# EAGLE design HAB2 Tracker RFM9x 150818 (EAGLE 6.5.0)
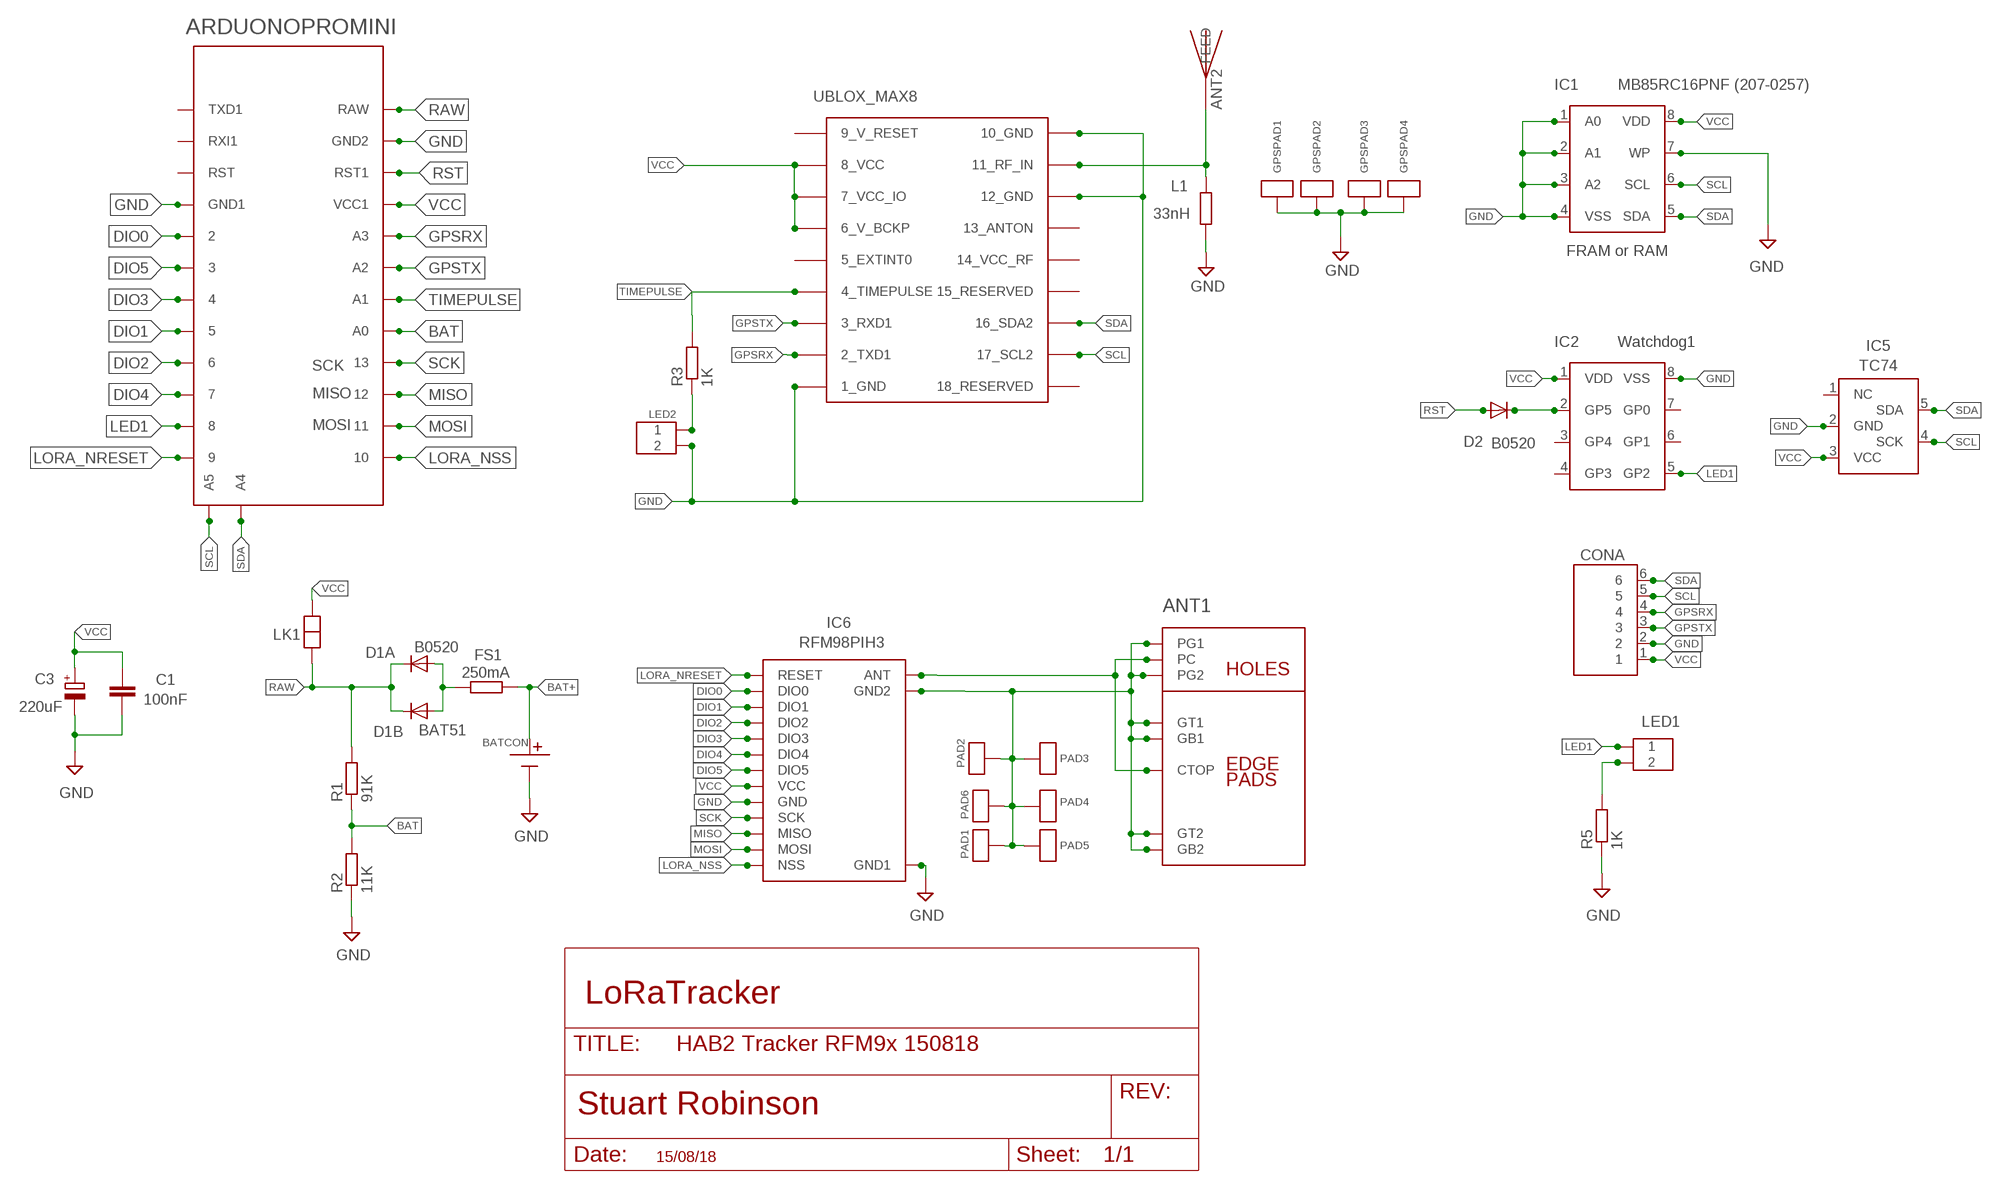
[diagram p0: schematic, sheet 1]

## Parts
ANT1  CUSTOMSMA  [CUSTOMSMA]
ANT2  JTI_ANTENNA-1575AT43A40  [JTI_ANTENNA-1575AT43A40]
BATCON  BATCON  [BATCON]
C1  100nF  C-EUC1206  [C1206]
C3  220uF  CPOL-EUSMCC  [SMC_C]
CONA  6X1  [6X1]
D1A  B0520  DIODE-SOD123  [SOD123]
D1B  BAT51  PIHDIODE  [PIHDIODE]
D2  B0520  DIODE-SOD123  [SOD123]
FS1  250mA  R-EU_R1206  [R1206]
GPSPAD1  ANTPAD2  [ANTPAD2]
GPSPAD2  ANTPAD2  [ANTPAD2]
GPSPAD3  ANTPAD2  [ANTPAD2]
GPSPAD4  ANTPAD2  [ANTPAD2]
IC1  MB85RC16PNF (207-0257)  24L256  [SOIC_2]
IC2  Watchdog1  12F1840_SOIC  [SOIC_2]
IC3  ARDUONOPROMINI  ARDUONOPROMINI_NOHEADER2  [ARDUINOPROMINDIP_NOHEADER2]
IC5  TC74  [SOT23-5]
IC6  RFM98PIH3  [RFM98PIH3]
L1  33nH  R-EU_R0603  [R0603]
LED1  2PIN  [2PIN]
LED2  2PIN  [2PIN]
LK1  2PADLINKLARGE  [2PADLINKLARGE]
PAD1  ANTPAD2  [ANTPAD2]
PAD2  ANTPAD2  [ANTPAD2]
PAD3  ANTPAD2  [ANTPAD2]
PAD4  ANTPAD2  [ANTPAD2]
PAD5  ANTPAD2  [ANTPAD2]
PAD6  ANTPAD2  [ANTPAD2]
R1  91K  R-EU_M1206  [M1206]
R2  11K  R-EU_M1206  [M1206]
R3  1K  R-EU_M1206  [M1206]
R5  1K  R-EU_M1206  [M1206]
UBLOX_MAX8  UBLOX_MAX  [UBLOX_MAX]

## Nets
ANT: ANT1.CTOP ANT1.PC IC6.ANT
BAT: IC3.A0 R1.1 R2.2
BAT+ [VDD]: D1A.A D1B.A FS1.2
DIO0: IC3.2 IC6.DIO0
DIO1: IC3.5 IC6.DIO1
DIO2: IC3.6 IC6.DIO2
DIO3: IC3.4 IC6.DIO3
DIO4: IC3.7 IC6.DIO4
DIO5: IC3.3 IC6.DIO5
GND [POWER]: ANT1.G1 ANT1.G2 ANT1.GB1 ANT1.GB2 ANT1.GT1 ANT1.GT2 BATCON.P$2(-) C1.2 C3.- CONA.2 GPSPAD1.P$1 GPSPAD2.P$1 GPSPAD3.P$1 GPSPAD4.P$1 IC1.1(A0) IC1.2(A1) IC1.3(A2) IC1.4(VSS) IC1.7(WP) IC2.8(VSS) IC3.GND1 IC3.GND2 IC5.2(GND) IC6.GND IC6.GND1 IC6.GND2 L1.1 LED2.P$2 PAD1.P$1 PAD2.P$1 PAD3.P$1 PAD4.P$1 PAD5.P$1 PAD6.P$1 R2.1 R5.1 UBLOX_MAX8.1_GND UBLOX_MAX8.10_GND UBLOX_MAX8.12_GND
GPSRX: CONA.4 IC3.A3 UBLOX_MAX8.2_TXD1
GPSTX: CONA.3 IC3.A2 UBLOX_MAX8.3_RXD1
LED1: IC2.5(GP2) IC3.8 LED1.P$1
LORA_NRESET: IC3.9 IC6.RESET
LORA_NSS: IC3.10 IC6.NSS
MISO: IC3.12 IC6.MISO
MOSI: IC3.11 IC6.MOSI
N$2 [POWER]: BATCON.P$1(+) FS1.1
N$3: D2.C IC2.2(GP5)
N$19: LED2.P$1 R3.1
N$41: LED1.P$2 R5.2
RAW [VDD]: D1A.C D1B.K IC3.RAW LK1.P$2 R1.2
RFIN: ANT2.FEED L1.2 UBLOX_MAX8.11_RF_IN
RST: D2.A IC3.RST2(RST1)
SCK: IC3.13 IC6.SCK
SCL: CONA.5 IC1.6(SCL) IC3.A5 IC5.4(SCK) UBLOX_MAX8.17_SCL2
SDA: CONA.6 IC1.5(SDA) IC3.A4 IC5.5(SDA) UBLOX_MAX8.16_SDA2
TIMEPULSE: IC3.A1 R3.2 UBLOX_MAX8.4_TIMEPULSE
VCC [VDD]: C1.1 C3.+ CONA.1 IC1.8(VDD) IC2.1(VDD) IC3.VCC1 IC5.3(VCC) IC6.VCC LK1.P$1 UBLOX_MAX8.6_V_BCKP UBLOX_MAX8.7_VCC_IO UBLOX_MAX8.8_VCC
Unconnected: IC2.3(GP4) IC2.4(GP3) IC2.6(GP1) IC2.7(GP0) IC3.RST IC3.RXI1 IC3.TXD1 IC5.1(NC) UBLOX_MAX8.5_EXTINT0 UBLOX_MAX8.13_ANTON UBLOX_MAX8.14_VCC_RF UBLOX_MAX8.15_RESERVED UBLOX_MAX8.18_RESERVED

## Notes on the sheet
- FRAM or RAM
- SCK
- MISO
- MOSI
- LoRaTracker
- 15/08/18

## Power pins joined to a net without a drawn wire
9_V_RESET: UBLOX_MAX8.9_V_RESET

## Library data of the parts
ANT1 = con-coax:CUSTOMSMA
ANT2 = Ava2:JTI_ANTENNA-1575AT43A40
BATCON = LMA2:BATCON
C1 = resistor:C-EU: CAPACITOR, European symbol
C3 = resistor:CPOL-EU: POLARIZED CAPACITOR, European symbol
CONA = My_Pin_Headers:6X1
D1A D2 = diode:DIODE-: DIODE
D1B = LMA2:PIHDIODE
FS1 L1 R1-R3 R5 = resistor:R-EU_: RESISTOR, European symbol
GPSPAD1-GPSPAD4 PAD1-PAD6 = LMA2:ANTPAD2
IC1 = LMA2:24L256
IC2 = LMA2:12F1840_SOIC
IC3 = LMA2:ARDUONOPROMINI_NOHEADER2
IC5 = LMA2:TC74
IC6 = LMA2:RFM98PIH3
LED1 LED2 = LMA2:2PIN
LK1 = LMA2:2PADLINKLARGE
UBLOX_MAX8 = Ava2:UBLOX_MAX: UBLOX MAX

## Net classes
0 default: width 0.152 mm
1 POWER: width 0.635 mm
2 VDD: width 0.635 mm
3 gpspower: width 0.635 mm

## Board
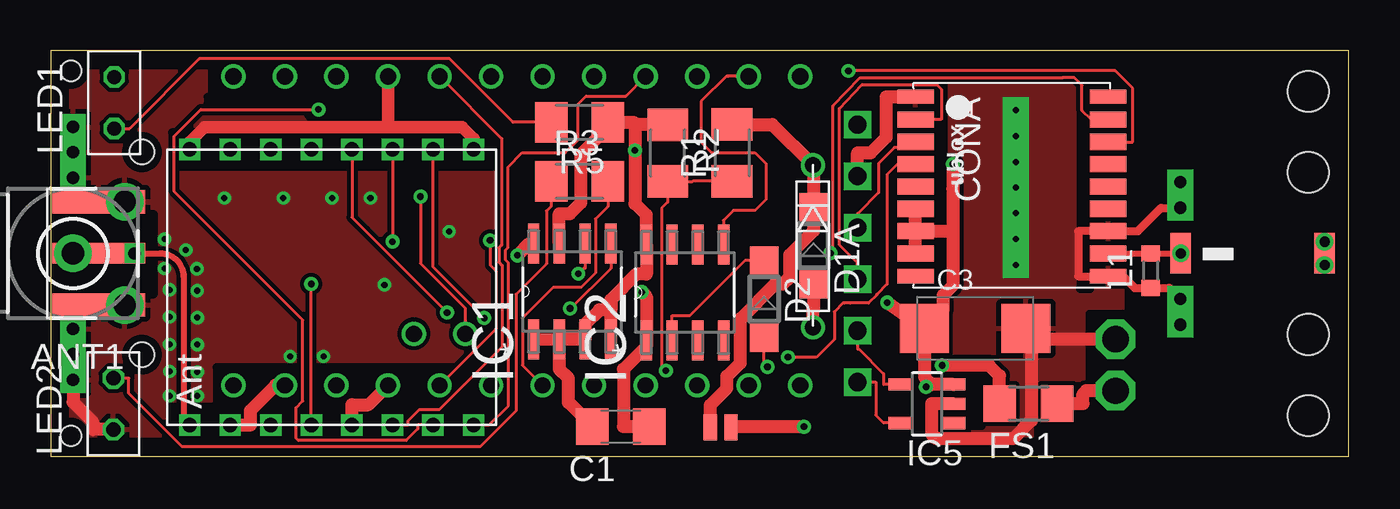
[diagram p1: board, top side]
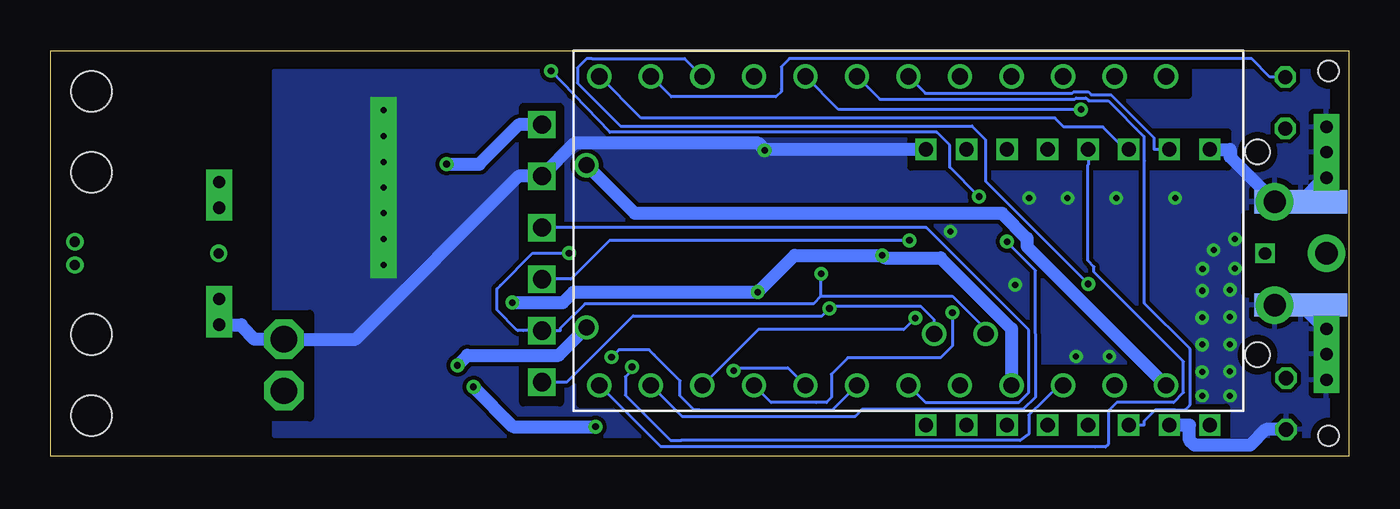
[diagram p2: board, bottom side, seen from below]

Size 64 x 20 mm. Coordinates in mm from the lower left corner, seen from the top.
Outline: 0,0 64,0 64,20 0,20 0,0
Copper layers (1*16): Top 0.0356mm / dielectric 1.5011mm / Bottom 0.0356mm
Design rules "LaenPCBOrder *": minimum track width 6mil, minimum drill 13mil, track to track 6mil, track to pad 6mil, pad to pad 6mil, via to via 6mil, smd to smd 6mil, copper to edge 15mil, drill to drill 6mil, minimum pad ring 7mil, minimum via ring 7mil, stop-mask expansion 4mil, vias tented up to drill 1000mil, thermal gap 10mil
Holes 2 mm at 62,2 62,6 62,18 62,14
Holes 1 mm at 1,1 1,19
Holes 1.2 mm at 4.5,15 4.5,5
tRestrict: area 56.5,0 to 63.9,19.9; area 53.1,7 to 55.1,14.8; area 50.8,8.2 to 51.2,18.4; area 43.6,8.2 to 44,18.4; area 6,14.3 to 22.1,16; area 5.9,0.7 to 21.9,2.4; area 22.8,0.9 to 41,17.9; area 7.9,17.8 to 38.4,19.9; area 0.1,8 to 5.1,11.9; area 40.9,14.8 to 41.7,18.2; area 12.9,16.7 to 13.6,17.4; area 8.2,2.6 to 37.9,4.4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
bRestrict: area 56.5,0.2 to 63.9,19.9; area 0.1,8 to 5.1,11.9; area 6.1,0.7 to 21.6,2.4; area 6,14.3 to 21.6,16; area 51.2,1.9 to 53.8,7; area 8.1,2.6 to 37.9,4.3; area 7.9,17.8 to 38.4,19.8; area 38.9,2.6 to 40.7,17.2

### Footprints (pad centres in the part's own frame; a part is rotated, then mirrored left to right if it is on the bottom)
CUSTOMSMA = smd 4.572 x 1.016: CTOP -1.27,0 | drill 1.1 pad 1.85: G1 -2.55,2.55; G2 -2.55,-2.55; PC 0,0 | smd 4.572 x 1.143 bottom: GB1 -1.27,2.54; GB2 -1.27,-2.54 | smd 4.572 x 1.143: GT1 -1.27,2.54; GT2 -1.27,-2.54
JTI_ANTENNA-1575AT43A40 = smd 1 x 2: FEED -3.175,0; NC 3.925,0
BATCON = drill 1.3 octagon: P$1 0,1.27; P$2 0,-1.27
C1206 = smd 1.6 x 1.8: 1 -1.4,0; 2 1.4,0
SMC_C = smd 2.4 x 2.4: + -2.5,0; - 2.5,0
6X1 = drill 0.9 square: 1 -6.35,0; 2 -3.81,0; 3 -1.27,0; 4 1.27,0; 5 3.81,0; 6 6.35,0
SOD123 = smd 1.4 x 1.4: A 1.9,0; C -1.9,0
PIHDIODE = drill 0.8: A 3,0; K -5,0
R1206 = smd 1.6 x 1.803: 1 -1.422,0; 2 1.422,0
ANTPAD2 = drill 0.6 pad 1.27 square: P$1 0,0
SOIC_2 = smd 1.981 x 0.559: 1 -2.362,1.905; 2 -2.362,0.635; 3 -2.362,-0.635; 4 -2.362,-1.905; 5 2.362,-1.905; 6 2.362,-0.635; 7 2.362,0.635; 8 2.362,1.905
ARDUINOPROMINDIP_NOHEADER2 = drill 0.8: 2 -7.62,-13.97; 3 -7.62,-16.51; 4 -7.62,-19.05; 5 -7.62,-21.59; 6 -7.62,-24.13; 7 -7.62,-26.67; 8 -7.62,-29.21; 9 -7.62,-31.75; 10 7.62,-31.75; 11 7.62,-29.21; 12 7.62,-26.67; 13 7.62,-24.13; A0 7.62,-21.59; A1 7.62,-19.05; A2 7.62,-16.51; A3 7.62,-13.97; A4 5.08,-15.24; A5 5.08,-12.7; GND1 -7.62,-11.43; GND2 7.62,-6.35; RAW 7.62,-3.81; RST -7.62,-8.89; RST2 7.62,-8.89; RXI1 -7.62,-6.35; TXD1 -7.62,-3.81; VCC1 7.62,-11.43
SOT23-5 = smd 0.6 x 1.2: 1 -0.95,-1.306; 2 0,-1.306; 3 0.95,-1.306; 4 0.95,1.306; 5 -0.95,1.306
RFM98PIH3 = drill 0.7 pad 1.016 square: ANT -6.8,6.23; DIO0 -6.8,-3.77; DIO1 -6.8,-5.77; DIO2 -6.8,-7.77; DIO3 -6.8,2.23; DIO4 -6.8,0.23; DIO5 6.8,4.23; GND -6.8,4.23; GND1 6.8,6.23; GND2 6.8,-7.77; MISO 6.8,-5.77; MOSI 6.8,-3.77; NSS 6.8,0.23; RESET 6.8,2.23; SCK 6.8,-1.77; VCC -6.8,-1.77
R0603 = smd 0.8 x 0.9: 1 -0.85,0; 2 0.85,0
2PIN = drill 0.7 octagon: P$1 0,1.27; P$2 0,-1.27
2PADLINKLARGE = smd 1.27 x 0.66: P$1 0,0.46; P$2 0,-0.56
M1206 = smd 1.6 x 2: 1 -1.4,0; 2 1.4,0
UBLOX_MAX = smd 1.8 x 0.7: 1_GND 4.95,-4.475; 9_V_RESET 4.95,4.375; 10_GND -4.55,4.375; 18_RESERVED -4.55,-4.475 | smd 1.8 x 0.8: 2_TXD1 4.95,-3.35; 3_RXD1 4.95,-2.25; 4_TIMEPULSE 4.95,-1.15; 5_EXTINT0 4.95,-0.05; 6_V_BCKP 4.95,1.05; 7_VCC_IO 4.95,2.15; 8_VCC 4.95,3.25; 11_RF_IN -4.55,3.25; 12_GND -4.55,2.15; 13_ANTON -4.55,1.05; 14_VCC_RF -4.55,-0.05; 15_RESERVED -4.55,-1.15; 16_SDA2 -4.55,-2.25; 17_SCL2 -4.55,-3.35

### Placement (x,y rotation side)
ANT1  1.1,10 180 top
ANT2  58.88,10 0 top
BATCON  52.5,4.49 180 top
C1  28.11,1.45 180 top
C3  45.58,6.3 0 top
CONA  39.78,10 270 top
D1A  37.61,10.38 270 top
D1B  37.58,9.35 270 top
D2  35.17,7.75 270 top
FS1  48.2,2.59 180 top
GPSPAD1  55.7,13.51 0 top
GPSPAD2  55.7,6.48 0 top
GPSPAD3  55.7,7.75 0 top
GPSPAD4  55.7,12.25 0 top
IC1  25.71,8.12 90 top
IC2  31.27,8.07 90 top
IC3  5.2,11.11 270 bottom
IC5  43.2,2.58 90 top
IC6  13.08,8.33 90 top
L1  54.23,9.15 90 top
LED1  3.13,17.43 0 top
LED2  3.09,2.58 0 top
LK1  33.08,1.42 270 top
PAD1  1.1,3.76 0 top
PAD2  1.1,5.03 0 top
PAD3  1.1,6.28 0 top
PAD4  1.1,13.73 0 top
PAD5  1.1,14.99 0 top
PAD6  1.1,16.24 0 top
R1  33.59,14.96 90 top
R2  30.42,14.95 270 top
R3  26.07,13.55 0 top
R5  26.07,16.47 180 top
UBLOX_MAX8  47.59,13.25 180 top

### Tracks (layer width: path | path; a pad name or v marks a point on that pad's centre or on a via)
ANT  (via drill 0.6)
  Top 0.152: ANT1.CTOP ANT1.PC | 5.38,10 v4.13,10
  Top 0.305: ANT1.CTOP v4.13,10 5.38,10 5.4,10 arc-90 6.55,8.85 6.55,1.83 arc90 IC6.ANT
BAT  (via drill 0.33 pad 0.69)
  Top 0.152: R1.1 31.66,13.56 31.65,13.55 R2.2 30.42,12.52 30.13,12.23 30.13,4.42 v30.33,4.21
  Bottom 0.152: v30.33,4.21 30.18,4.36 27.66,4.36 IC3.A0
BAT+  (via drill 0.33 pad 0.69)
  Top 0.635: FS1.2 46.78,3.96 46.27,4.47 v43.95,4.47 | D1A.A 37.61,7.31 37.58,7.28 D1B.A
  Bottom 0.635: v43.95,4.47 43.45,4.97 38.96,4.97 D1B.A
DIO0
  Top 0.152: IC3.2 22.24,15.66 22.24,10.41 22.1,10.27 22.1,9.57 22.26,9.41 22.26,5.39 19.16,2.29 18.17,2.29 17.61,1.72 17.61,1.53 IC6.DIO0
DIO1  (via drill 0.33 pad 0.69)
  Top 0.152: v13.2,17.1 7.4,17.1 6.09,15.79 6.09,13.05 12.43,6.71 12.43,2.72 12.09,2.38 12.09,0.88 12.2,0.77 17.53,0.77 18.09,1.34 18.09,1.53 IC6.DIO1
  Bottom 0.152: v13.2,17.1 25.16,17.1 IC3.5
DIO2
  Top 0.152: IC6.DIO2 21.61,1.53 22.57,2.49 22.57,9.54 22.43,9.67 22.43,10.18 22.54,10.28 22.54,13.54 22.54,14.25 23.25,14.96 25.36,14.96 26,15.6 26,17.36 26.4,17.76 28.36,17.76 IC3.6
DIO3
  Bottom 0.152: IC3.4 23.12,17.6 13.51,17.6 13.44,17.67 12.97,17.67 12.82,17.52 11.86,17.52 10.09,15.76 10.09,14.57 10.08,14.56 10.08,7.54 7.85,5.31 7.85,5.3 7.82,5.27 7.82,2.53 7.84,2.51 8.06,2.29 8.56,2.29 9.53,2.29 10.09,1.72 10.09,1.53 IC6.DIO3
DIO4  (via drill 0.33 pad 0.69)
  Top 0.152: IC6.DIO4 v12.85,8.49
  Bottom 0.152: v12.85,8.49 12.85,8.5 17.89,13.55 17.89,15.59 18.36,16.05 | 18.36,16.05 18.58,16.28 | IC3.7 32.74,19.61 37.31,19.61 37.55,19.61 37.56,19.61 37.57,19.61 38.03,19.15 38.03,18.4 35.91,16.28 18.58,16.28 | 18.58,16.28 18.36,16.05
DIO5
  Bottom 0.152: IC3.3 20.88,17.9 13.64,17.9 13.57,17.97 12.84,17.97 12.69,17.83 11.72,17.83 9.61,15.71 9.61,15.13 IC6.DIO5
GND  (via drill 0.3, 0.3 pad 1.27, 0.33 pad 0.69)
  Top 0.406: GPSPAD1.P$1 GPSPAD4.P$1 54.74,12.24 53.6,11.1 UBLOX_MAX8.12_GND 50.66,11.1 50.66,8.87 UBLOX_MAX8.10_GND 52.87,8.88 53.45,8.29 L1.1 55.15,8.3 GPSPAD3.P$1 GPSPAD2.P$1
  Top 0.61: IC6.GND1 6.85,15.49 7.6,16.23 16.54,16.23 | 16.54,16.23 19.83,16.23 | 19.83,16.23 19.86,16.23 | 19.83,16.23 20.29,16.23 20.85,15.67 IC6.GND2 | IC3.GND1 16.63,16.32 16.54,16.23 | IC1.1 IC1.2
  Top 0.635: 48.35,5.76 48.35,1.75 47.46,0.86 43.65,0.86 43.44,1.07 43.44,2.58 IC5.2 | C3.- 48.35,6.03 48.35,5.76 | 48.35,5.76 51.05,5.76 BATCON.P$2 | IC1.7 25.07,11.94 25.59,11.94 26.13,12.49 26.13,14.88 27.73,16.47 | R5.1 27.73,16.47 | 27.73,16.47 28.11,16.47 28.74,16.47 28.86,16.35 | 28.86,16.35 28.8,16.29 v28.8,15.08 28.8,12.46 29.36,11.89 IC2.8 29.36,8.97 28.87,8.97 27.61,7.71 27.61,7.22 | R2.1 28.86,16.35 | LED2.P$2 2.09,1.31 2.09,1.66 1.1,2.65 PAD1.P$1 | CONA.2 39.78,14.96 40.42,14.96 41.18,15.71 41.18,17.73 41.27,17.73 arc90 41.37,17.73 UBLOX_MAX8.1_GND arc-90 UBLOX_MAX8.1_GND | IC1.4 27.61,7.22 | IC6.GND 9.85,1.53 9.85,2.25 11.09,3.49 IC3.GND2 | 27.61,7.22 27.05,7.22 26.34,6.51 IC1.3 IC1.2 25.07,4.3 25.52,3.85 25.52,2.64 C1.2 | ANT1.G1 ANT1.GB1 | ANT1.G2 ANT1.GB2
  Bottom 0.635: GPSPAD2.P$1 54.59,6.48 54.59,6.41 53.95,5.76 BATCON.P$2 48.98,5.76 40.92,13.81 CONA.2 38.16,15.43 29.1,15.43 28.8,15.13 | 1.28,6.28 1.28,6.37 ANT1.GB1 ANT1.G1 | ANT1.GB2 ANT1.G2 5.85,14.75 5.85,15.13 IC6.GND1 | ANT1.GB2 2.21,12.71 | 1.28,6.28 1.14,6.13 1.1,6.13 PAD2.P$1 PAD1.P$1 | PAD3.P$1 1.28,6.28 | IC6.GND 7.85,1.53 7.85,0.78 7.6,0.53 4.87,0.53 4.09,1.31 LED2.P$2 | 28.8,15.13 v28.8,15.08 | IC6.GND2 28.8,15.13 | PAD6.P$1 PAD5.P$1 1.1,13.88 PAD4.P$1 1.18,13.73 ANT1.GB2
  other vias: 5.61,9.25 5.61,10.7 7.23,6.83 5.86,8.2 7.23,5.5 5.86,6.86 7.23,4.15 5.86,5.51 7.22,8.16 5.87,4.18 7.23,2.97 5.86,2.97 6.66,10.17 7.21,9.24 47.59,13.25 47.59,14.51 47.59,15.79 47.59,17.06 47.59,11.98 47.59,10.71 47.59,9.43 8.56,12.73 11.47,12.73 13.87,12.73 11.81,4.92 13.45,4.92 15.76,12.73 16.45,8.45 19.64,11.08
  pour Top (isolate 0.2): 1,19 53,19 53,1 1,1
  pour Bottom (isolate 0.2): 1,19 53,19 53,1 1,1
GPSRX  (via drill 0.33 pad 0.69)
  Top 0.152: UBLOX_MAX8.2_TXD1 43.72,16.6 43.91,16.61 43.91,18.11 43.69,18.33 40.01,18.33 38.88,17.14 38.88,10.42 39.67,9.63 39.78,9.63 CONA.4 | v21.66,10.64 21.66,9.42 21.96,9.13 21.96,6.28 IC3.A3
  Bottom 0.152: v21.66,10.64 36.44,10.64 38.36,8.73 CONA.4
GPSTX
  Top 0.152: UBLOX_MAX8.3_RXD1 42.12,15.5 42.03,15.5 41.76,15.23 41.58,15.23 41.58,15.2 40.81,14.43 40.81,12.99 39.79,11.97 CONA.3
  Bottom 0.152: IC3.A2 20.88,2.66 16.26,2.66 15.78,3.14 15.78,6.21 20.84,11.27 CONA.3
LED1
  Top 0.152: IC3.8 33.8,18.73 33.4,18.73 33.39,18.74 33.31,18.74 32.07,17.5 32.07,15.49 32.59,14.97 34.53,14.97 34.72,14.97 35.27,14.42 35.27,12.66 34.73,12.12 33.66,12.12 33.17,11.63 IC2.5
  Bottom 0.152: LED1.P$1 3.89,18.7 4.79,19.61 27.09,19.61 27.59,19.61 27.98,19.21 27.98,18.11 27.98,17.99 28.25,17.72 33.4,17.72 IC3.8
LORA_NRESET
  Bottom 0.152: IC3.9 34.89,16.67 14.49,16.67 14.06,16.24 12.12,16.24 11.01,15.13 IC6.RESET
LORA_NSS
  Bottom 0.152: IC6.NSS 12.85,14.37 12.86,14.36 12.86,9.64 12.56,9.34 12.56,9.07 8.15,4.66 8.15,3.14 8.63,2.66 8.66,2.66 11.1,2.66 11.43,2.66 11.86,2.23 11.86,0.59 12,0.45 12.52,0.45 12.52,0.46 33.92,0.46 IC3.10
MISO  (via drill 0.33 pad 0.69)
  Top 0.152: v21.37,6.8 18.85,9.33 IC6.MISO
  Bottom 0.152: v21.37,6.8 21.93,6.24 29.12,6.24 IC3.12
MOSI  (via drill 0.33 pad 0.69)
  Top 0.152: IC6.MOSI v16.85,10.58
  Bottom 0.152: IC3.11 32.88,1.96 24.33,1.96 23.99,2.33 16.04,2.33 15.43,2.92 15.45,9.16 16.85,10.56 v16.85,10.58
N$2
  Top 0.635: FS1.1 50.89,2.59 50.89,3.06 51.05,3.22 BATCON.P$1
N$3
  Top 0.152: D2.C 34.24,9.65 31.52,6.93 30.64,6.93 IC2.2
N$4  (via drill 0.5 pad 0.69)
  other vias: 62.81,10.57
N$5  (via drill 0.5 pad 0.69)
  other vias: 62.81,9.43
N$19
  Top 0.152: LED2.P$1 3.85,3.85 3.85,3.09 6.47,0.47 21.18,0.47 22.94,2.23 22.94,7.98 24.44,9.48 24.44,12.09 24.67,12.32 R3.1
N$41
  Top 0.152: LED1.P$2 3.89,16.16 7.32,19.6 19.67,19.6 22.8,16.47 R5.2
RAW
  Top 0.635: LK1.P$2 32.52,2.52 33.34,3.35 33.34,3.93 34,4.59 34,6.78 35.7,8.48 36.07,8.48 36.44,8.85 36.44,9.94 37.61,11.11 D1A.C 37.61,14.32 D1B.K 35.57,16.36 R1.2
  Bottom 0.635: D1B.K 35.21,11.98 17.1,11.98 15.86,10.74 15.86,10.34 IC3.RAW
RFIN  (via drill 0.5 pad 0.69)
  Top 0.152: ANT2.FEED | ANT2.FEED v55.72,10
  Top 0.305: UBLOX_MAX8.11_RF_IN L1.2 ANT2.FEED
RST  (via drill 0.33 pad 0.69)
  Top 0.152: v35.34,4.4 35.17,4.57 D2.A
  Bottom 0.152: IC3.RST2 14.27,3.49 15.78,2.02 15.78,1.1 16.21,0.77 32.91,0.77 32.91,0.78 33.45,0.78 35.67,3 35.67,3.91 35.34,4.24 v35.34,4.4
SCK  (via drill 0.33 pad 0.69)
  Top 0.152: IC6.SCK 14.85,11.77 v19.54,7.08
  Bottom 0.152: v19.54,7.08 19.54,5.69 19.54,5.44 20.13,4.85 24.7,4.85 25.51,4.04 25.51,2.89 25.75,2.65 26.26,2.65 26.27,2.65 28.49,2.65 IC3.13
SCL  (via drill 0.33 pad 0.69)
  Top 0.152: v38.44,10.01 38.57,10.14 38.57,17.28 39.89,18.66 49.88,18.66 49.89,18.66 50.48,18.66 50.85,18.29 50.85,17.05 51.3,16.6 51.61,16.6 UBLOX_MAX8.17_SCL2 | IC5.4 41.06,3.53 41.06,4.06 39.84,5.29 39.78,5.29 CONA.5 | v26.01,8.99 26.28,9.26 26.34,9.26 IC1.6
  Bottom 0.152: 26.01,7.89 26.39,7.52 37.66,7.52 38.88,6.3 38.88,6.19 CONA.5 40.69,6.19 40.98,6.19 40.98,6.21 41,6.21 42,7.21 42,8.25 41.83,8.42 | 26.01,7.89 19.55,7.89 17.9,6.25 IC3.A5 | 26.01,7.89 v26.01,8.99 | v38.44,10.01 40.24,10.01 41.83,8.42 | 41.83,8.42
SDA  (via drill 0.33 pad 0.69)
  Top 0.152: IC5.5 41.06,1.63 40.68,2.01 40.68,3.65 CONA.6 | v18.23,12.81 18.23,9.51 20.44,7.3 IC3.A4 | v39.34,19 52.49,19 53.35,18.15 53.35,15.5 UBLOX_MAX8.16_SDA2 | v25.6,7.28 25.64,7.28 27.61,9.26 IC1.5
  Bottom 0.152: v18.23,12.81 19.67,14.25 19.67,15.33 20.31,15.97 36.43,15.97 v39.34,19 | CONA.6 38.55,3.65 35.28,6.92 25.97,6.92 v25.6,7.28 25.5,7.38 21.11,7.38 20.44,6.72 IC3.A4
TIMEPULSE  (via drill 0.33 pad 0.69)
  Top 0.152: R3.2 27.47,12.32 26.85,11.7 26.85,9.03 26.15,8.33 24.77,8.33 23.26,6.81 23.26,4.48 IC3.A1 | UBLOX_MAX8.4_TIMEPULSE 41.75,14.4 41.24,13.89 41.24,8.49 40.73,7.98 40.73,7.96 40.32,7.55 39.42,7.55 39.13,7.55 39.12,7.56 39.07,7.56 38.63,7.12 38.63,5.76 37.75,4.88 v36.35,4.88
  Bottom 0.152: IC3.A1 25.45,2.29 32.03,2.29 32.29,2.29 32.97,2.97 32.97,3.71 34.25,4.99 34.25,5 34.49,5.24 35.99,5.24 v36.35,4.88
VCC  (via drill 0.33 pad 0.69)
  Top 0.635: 43.36,3.61 43.44,3.53 IC5.3 | C3.+ 43.08,3.89 43.36,3.61 | 43.36,3.61 v43.16,3.41 | v29.14,8.09 29.36,7.86 IC2.1 29.36,5.4 28.24,4.28 28.24,1.45 C1.1 | IC6.VCC 14.85,2.53 15.67,2.53 IC3.VCC1 | IC1.8 23.59,10.48 v23.01,9.9 | v44.48,14.4 44.48,13.18 44.48,11.12 | 44.48,11.12 44.48,10.96 44.48,8.42 43.99,7.93 43.99,7.21 C3.+ | UBLOX_MAX8.8_VCC UBLOX_MAX8.7_VCC_IO | UBLOX_MAX8.7_VCC_IO UBLOX_MAX8.6_V_BCKP | v41.24,7.57 C3.+ | v37.13,1.45 33.54,1.45 LK1.P$1 | UBLOX_MAX8.7_VCC_IO 44.46,11.1 44.48,11.12
  Bottom 0.635: v43.16,3.41 41.2,1.45 v37.13,1.45 | CONA.1 40.92,16.35 42.88,14.4 v44.48,14.4 | v41.24,7.57 38.74,7.57 38.23,8.09 v29.14,8.09 27.32,9.9 v23.01,9.9 22.88,9.78 20.12,9.78 16.63,6.28 IC3.VCC1

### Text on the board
Notes_Bottom: - | + | BAT
Notes: A | 1 | LED1 | R5 | A | C | 150818 | R3 | R2 | R1 | UBLOX GPS | RFM9x | D1 | Stuart Robinson | L1 | ANT | IC1 | IC2 | 1 | 1 | D2 | + | C3 | - | - | A | FS1 | IC5 | + | LED2 | LK1 | C1 | 6 | BAT | C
